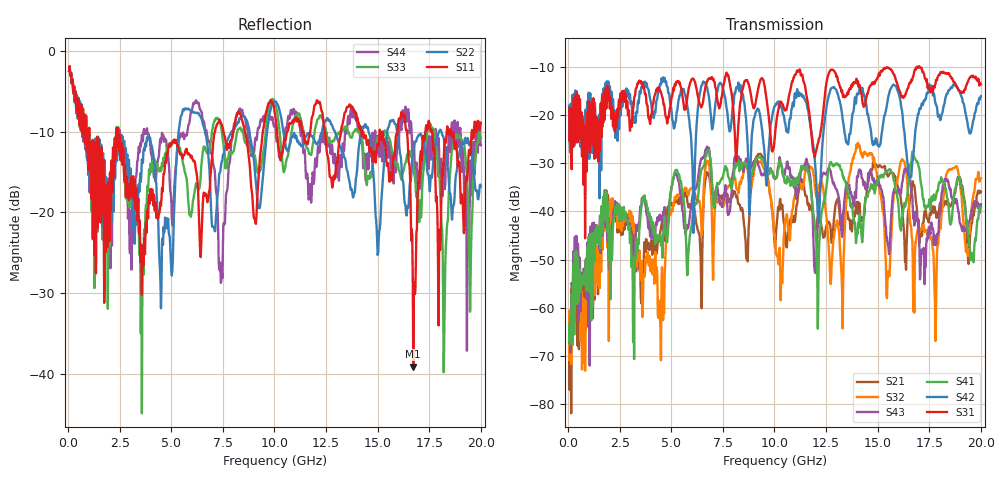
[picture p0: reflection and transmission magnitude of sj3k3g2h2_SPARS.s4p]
! FILE: E:\users\goganessyan\GBX_Backplane\FR408_backplane\1m_OUTBOUND_NEXT\sj3k3g2h2_SPARS.s4p
# MHZ S RI R 50.00
! FREQ  S11  S12  S13  S14
!  S21  S22  S23  S24
!  S31  S32  S33  S34
!  S41  S42  S43  S44
!  REAL  IMAG  REAL  IMAG  REAL  IMAG  REAL  IMAG
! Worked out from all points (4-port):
!   799 points, 50 MHz to 20 GHz, reference 50 ohm
!   strongest paths, dB at 50 MHz, 5.025 GHz, 10.03 GHz, 15.03 GHz, 20 GHz:
!     S31: -18.6, -16.1, -23.9, -12.1, -13.6
!     S42: -18.1, -20.0, -18.1, -26.2, -16.1
!     S41: -63.5, -34.7, -33.1, -33.0, -39.2
!     S43: -66.3, -34.7, -33.3, -33.8, -38.5
!     S32: -60.6, -39.5, -45.5, -34.0, -33.2
!     S21: -69.9, -38.7, -47.5, -30.5, -35.9
!   lowest |S11| = -39.1 dB at 16.73 GHz (marker M1), VSWR 1.02, Z = 50.4 - j1.03 ohm
!   |S11| at or under -10 dB: 1.027 GHz to 2.333 GHz (1.306 GHz wide, 77.7 % of centre); 2.431 GHz to 7.115 GHz (4.684 GHz wide, 98.1 % of centre); 18.56 GHz to 19.56 GHz (1.002 GHz wide, 5.26 % of centre)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
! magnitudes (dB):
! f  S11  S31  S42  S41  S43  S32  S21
! 50 MHz  -2.5  -18.6  -18.1  -63.5  -66.3  -60.6  -69.9
! 6.75 GHz  -18.8  -12.9  -14.6  -27.8  -26.8  -29.8  -32.2
! 12.1 GHz  -6.3  -26.0  -41.0  -64.4  -42.4  -36.4  -41.1
! 12.78 GHz  -16.4  -10.6  -14.4  -30.0  -33.1  -50.6  -46.5
! 14.05 GHz  -8.8  -13.0  -15.7  -42.4  -32.9  -25.8  -38.0
! 16.73 GHz  -39.1  -12.0  -28.6  -28.4  -41.5  -60.8  -34.5
! 20 GHz  -8.9  -13.6  -16.1  -39.2  -38.5  -33.2  -35.9
